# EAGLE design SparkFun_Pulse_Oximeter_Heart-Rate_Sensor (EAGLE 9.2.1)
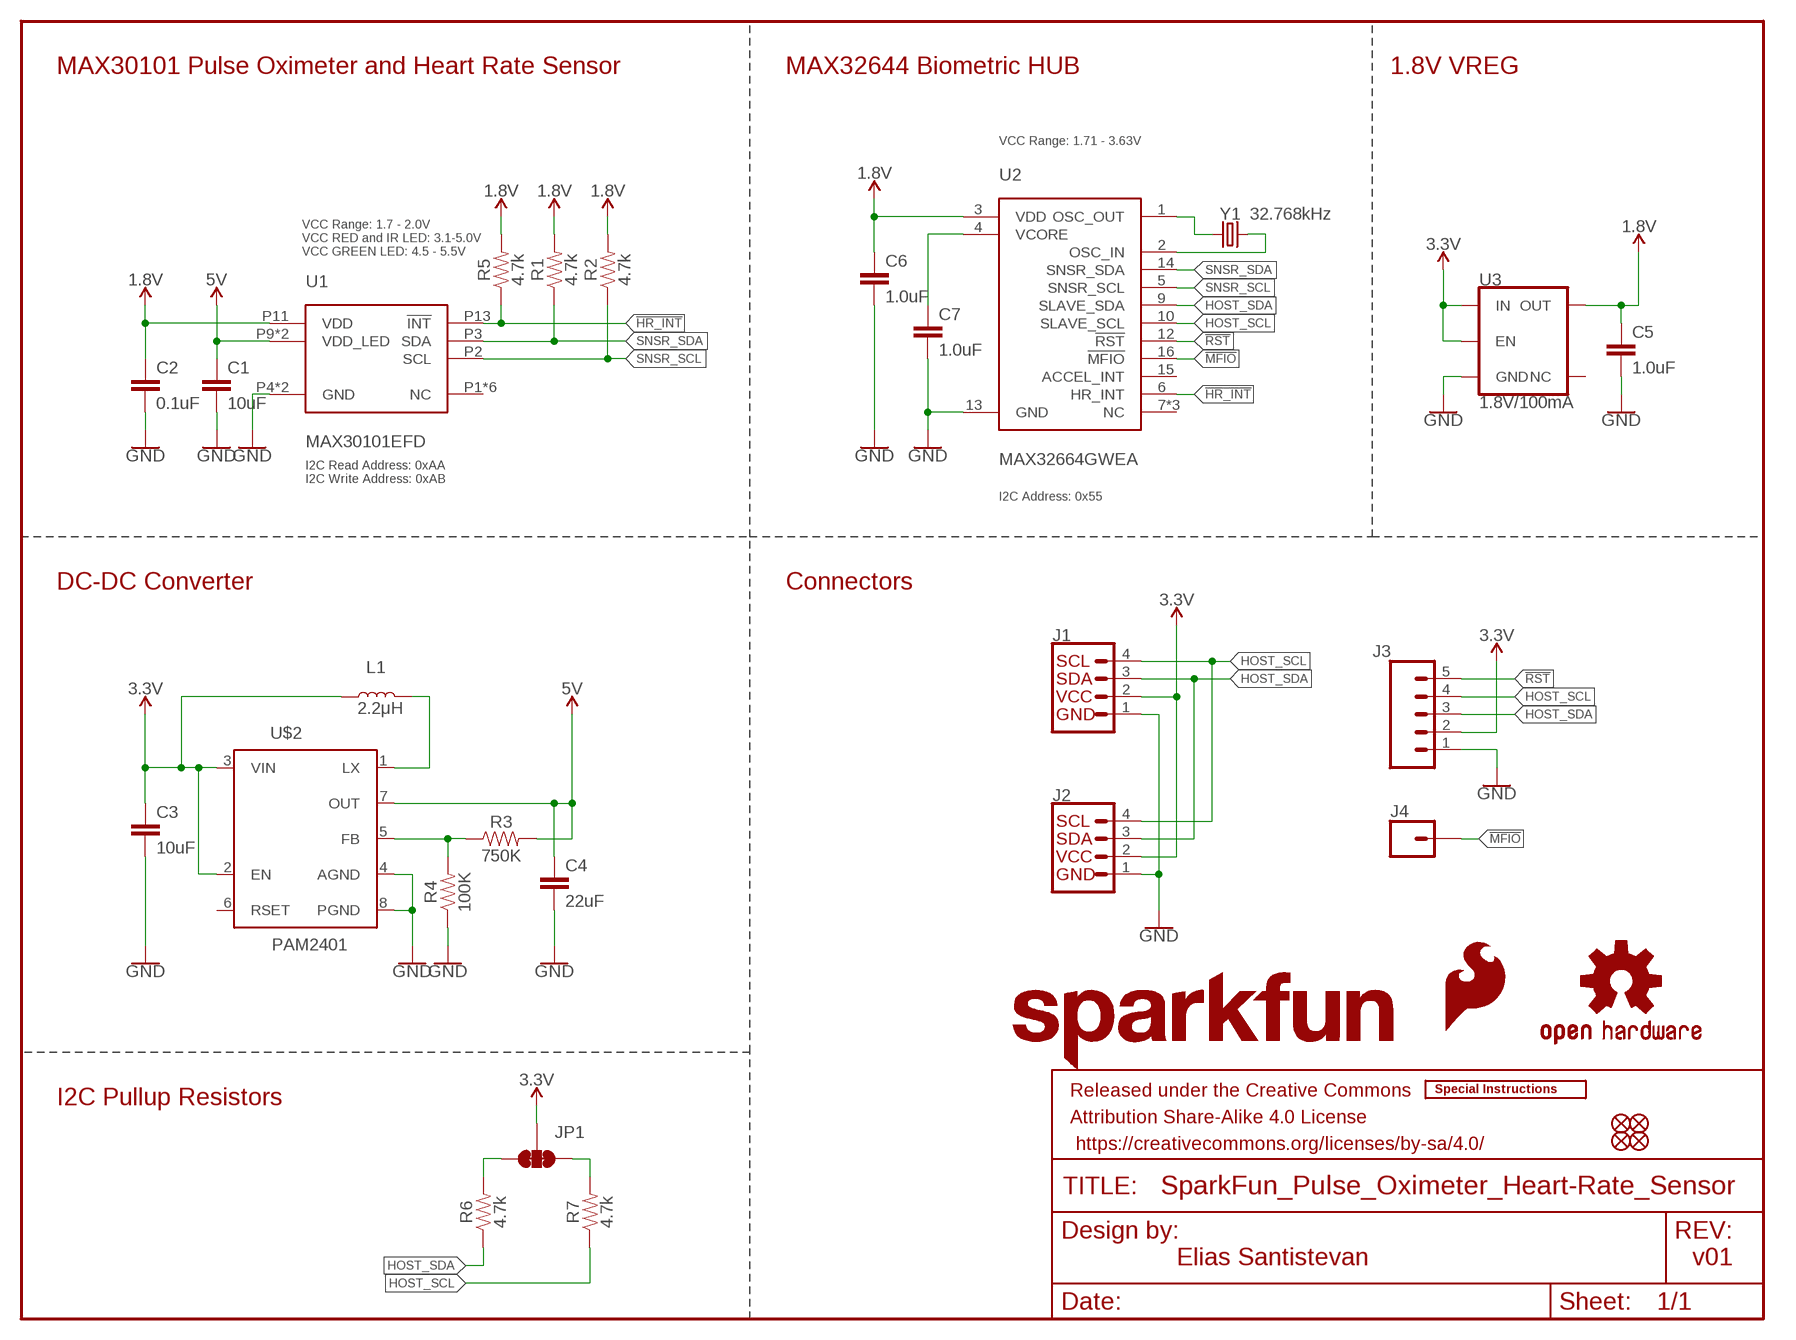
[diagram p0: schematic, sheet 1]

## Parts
C1  10uF  10UF-0603-6.3V-20%  [0603]
C2  0.1uF  0.1UF-0402-16V-10%  [0402]
C3  10uF  10UF-0603-6.3V-20%  [0603]
C4  22uF  22UF-0805-6.3V-20%  [0805]
C5  1.0uF  1.0UF-0603-16V-10%  [0603]
C6  1.0uF  1.0UF-0402-16V-10%  [0402]
C7  1.0uF  1.0UF-0402-16V-10%  [0402]
FD1  FIDUCIALUFIDUCIAL  [FIDUCIAL-MICRO]
FD2  FIDUCIALUFIDUCIAL  [FIDUCIAL-MICRO]
FD3  FIDUCIALUFIDUCIAL  [FIDUCIAL-MICRO]
FD4  FIDUCIALUFIDUCIAL  [FIDUCIAL-MICRO]
FRAME1  FRAME-LETTER  [CREATIVE_COMMONS]
J1  QWIIC_CONNECTORJS-1MM  [JST04_1MM_RA]
J2  QWIIC_CONNECTORJS-1MM  [JST04_1MM_RA]
J3  CONN_05NO_SILK  [1X05_NO_SILK]
J4  CONN_01PTH_NO_SILK_YES_STOP  [1X01_NO_SILK]
JP1  JUMPER-SMT_3_2-NC_TRACE_SILK  [SMT-JUMPER_3_2-NC_TRACE_SILK]
L1  2.2μH  2.2μH_SHIELDED_INDUCTOR  [0806]
LOGO1  SFE_LOGO_FLAME.1_INCH  [SFE_LOGO_FLAME_.1]
LOGO2  OSHW-LOGOMINI  [OSHW-LOGO-MINI]
LOGO3  SFE_LOGO_NAME.1_INCH  [SFE_LOGO_NAME_.1]
LOGO4  SPECIAL_INSTRUCTIONS-ORDERING  [ORDERING_INSTRUCTIONS]
R1  4.7k  4.7KOHM-0603-1/10W-1%  [0603]
R2  4.7k  4.7KOHM-0603-1/10W-1%  [0603]
R3  750K  750KOHM-0603-1/10W-1%  [0603]
R4  100K  100KOHM-0402-1/16W-1%  [0402]
R5  4.7k  4.7KOHM-0603-1/10W-1%  [0603]
R6  4.7k  4.7KOHM-0603-1/10W-1%  [0603]
R7  4.7k  4.7KOHM-0603-1/10W-1%  [0603]
U1  MAX30101EFD  [14_PIN_OESIP]
U2  MAX32664GWEA  [16_PIN_WLP]
U3  1.8V/100mA  V_REG_SP6214-1.8V  [SC70]
U$2  PAM2401  [MSOP8]
Y1  32.768kHz  CRYSTAL-32.768KHZSMD-3.2X1.5  [CRYSTAL-SMD-3.2X1.5MM]

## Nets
1.8V: C2.1 C5.1 C6.1 R1.2 R2.2 R5.2 U1.P11(VDD) U2.3(VDD) U3.5(OUT)
3.3V: C3.1 J1.2 J2.2 J3.2 JP1.2 L1.1 U3.1(IN) U3.3(EN) U$2.2(EN) U$2.3(VIN)
5V: C1.1 C4.1 R3.2 U1.P9(VDD_LED) U1.P10(VDD_LED) U$2.7(OUT)
!HR_INT: R5.1 U1.P13(!INT) U2.6(HR_INT)
!MFIO: J4.1 U2.16(!MFIO)
!RST: J3.5 U2.12(!RST)
GND: C1.2 C2.2 C3.2 C4.2 C5.2 C6.2 C7.2 J1.1 J2.1 J3.1 R4.1 U1.P4(GND) U1.P12(GND) U2.13(GND) U3.2(GND) U$2.4(AGND) U$2.8(PGND)
HOST_SCL: J1.4 J2.4 J3.4 R7.1 U2.10(SLAVE_SCL)
HOST_SDA: J1.3 J2.3 J3.3 R6.1 U2.9(SLAVE_SDA)
N$1: C7.1 U2.4(VCORE)
N$2: R3.1 R4.2 U$2.5(FB)
N$3: L1.2 U$2.1(LX)
N$4: JP1.3 R6.2
N$5: JP1.1 R7.2
N$6: U2.1(OSC_OUT) Y1.P$1
N$7: U2.2(OSC_IN) Y1.P$2
SNSR_SCL: R2.1 U1.P2(SCL) U2.5(SNSR_SCL)
SNSR_SDA: R1.1 U1.P3(SDA) U2.14(SNSR_SDA)
Unconnected: U1.P1(NC) U1.P5(NC) U1.P6(NC) U1.P7(NC) U1.P8(NC) U1.P14(NC) U2.7(NC) U2.8(NC) U2.11(NC) U2.15(ACCEL_INT) U3.4(NC) U$2.6(RSET)

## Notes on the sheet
- MAX30101 Pulse Oximeter and Heart Rate Sensor | MAX32644 Biometric HUB | 1.8V VREG
- VCC Range: 1.71 - 3.63V
- VCC Range: 1.7 - 2.0V
  VCC RED and IR LED: 3.1-5.0V
  VCC GREEN LED: 4.5 - 5.5V
- I2C Read Address: 0xAA
  I2C Write Address: 0xAB
- I2C Address: 0x55
- DC-DC Converter | Connectors
- I2C Pullup Resistors
- Elias Santistevan | v01

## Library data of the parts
C1 C3 = SparkFun-Capacitors:10UF: 10.0µF ceramic capacitors; PROD_ID: CAP-11015
C2 = SparkFun-Capacitors:0.1UF: 0.1µF ceramic capacitors; PROD_ID: CAP-12416
C4 = SparkFun-Capacitors:22UF: 22µF ceramic capacitors; PROD_ID: CAP-08402
C5 = SparkFun-Capacitors:1.0UF: 1µF ceramic capacitors; PROD_ID: CAP-00868
C6 C7 = SparkFun-Capacitors:1.0UF: 1µF ceramic capacitors; PROD_ID: CAP-12417
FD1-FD4 = SparkFun-Aesthetics:FIDUCIAL: Fiducial Alignment Points
FRAME1 = SparkFun-Aesthetics:FRAME-LETTER: Schematic Frame - Letter
J1 J2 = SparkFun-Connectors:QWIIC_CONNECTOR: SparkFun I2C Standard Qwiic Connector An SMD 1mm pitch JST connector makes it easy and quick (get it? Qwiic?) to connect I2C devices to each other. The Qwiic system enables fast and solderless connection between popular platforms and various sensors and actuators. We carry 200mm, 100mm, 50mm, and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; PROD_ID: CONN-13694
J3 = SparkFun-Connectors:CONN_05: Multi connection point. Often used as Generic Header-pin footprint for 0.1 inch spaced/style header connections On any of the 0.1 inch spaced packages, you can populate with these: Break Away Headers - Straight (PRT-00116) Break Away Male Headers - Right Angle (PRT-00553) Female Headers (PRT-00115)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
J4 = SparkFun-Connectors:CONN_01: Single connection point. Often used as Generic Header-pin footprint for 0.1 inch spaced/style header connections
JP1 = SparkFun-Jumpers:JUMPER-SMT_3_2-NC_TRACE: Normally closed trace jumper (2 of 2 connections) This jumper has a trace between all three pads so they are normally closed (NC). Use a razor knife to open the connection(s). For best results follow the IPC guidelines for cutting traces: Cutout at least 0.063 mm (0.005 in). Remove all loose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
L1 = SparkFun-Coils:2.2μH_SHIELDED_INDUCTOR: Murata 2.2uH Inductor; PROD_ID: NDUC-14257
LOGO1 = SparkFun-Aesthetics:SFE_LOGO_FLAME: SparkFun Flame Logo
LOGO2 = SparkFun-Aesthetics:OSHW-LOGO: Open-Source Hardware (OSHW) Logo
LOGO3 = SparkFun-Aesthetics:SFE_LOGO_NAME: SparkFun Font Logo
LOGO4 = SparkFun-Aesthetics:SPECIAL_INSTRUCTIONS: Special Ordering/Production Instructions Alert
R1 R2 R5-R7 = SparkFun-Resistors:4.7KOHM: 4.7kΩ resistor; PROD_ID: RES-07857
R3 = SparkFun-Resistors:750KOHM: 750Ω resistor; PROD_ID: RES-13768
R4 = SparkFun-Resistors:100KOHM: 100kΩ resistor; PROD_ID: RES-13495
U1 = SparkFun-IC-Special-Function:MAX30101EFD: MAX30101 High-Sensitivity Pulse Oximeter and Heart-Rate Sensor The MAX30101 is an integrated pulse oximetry and heart-rate monitor module. It includes internal LEDs, photodetectors, optical elements, and low-noise electronics with ambient light rejection. The MAX30101 provides a complete system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; PROD_ID: IC-14270
U2 = SparkFun-IC-Special-Function:MAX32664GWEA: Maxim MAX32664 Biometric Sensor Hub he MAX32664 is a sensor hub family with embedded firmware and algorithms for wearables. It seamlessly enables customer-desired sensor functionality, including communication with Maxim’s optical sensor solutions and delivering raw or calculated data to the outside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; PROD_ID: IC-14271
U3 = SparkFun-IC-Power:V_REG_SP6214: Voltage Regulator - SP6214 SP6214 Series SC-70-5 Micropower SC-70 100 mA CMOS LDO Regulator Datasheet SparkFun Products: MP3 Trigger SparkFun Particle Sensor Breakout; PROD_ID: VREG-08428
U$2 = SparkFun-IC-Power:PAM2401: PAM2401 - Boost PMIC Specifications: Up to 1A output current 0.9V to 4.75V Input Range 2.5V to 5.0V Adjustable Output Voltage Datasheet (Diodes inc.); PROD_ID: IC-13769
Y1 = SparkFun-Clocks:CRYSTAL-32.768KHZ: 32.768kHz Crystal; PROD_ID: XTAL-13062

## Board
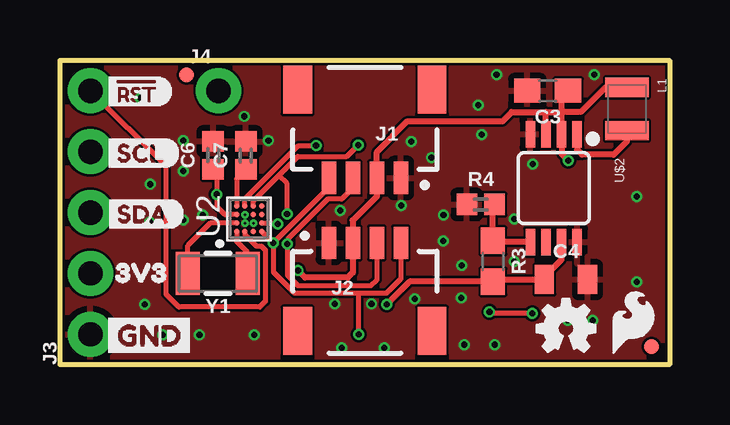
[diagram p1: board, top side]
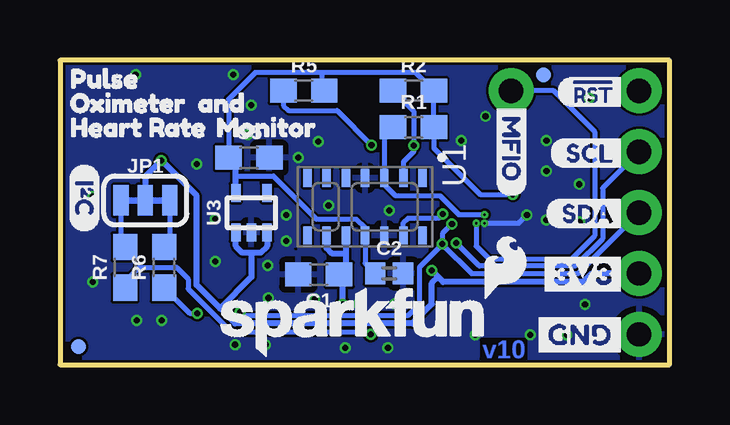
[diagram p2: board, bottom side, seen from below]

Size 25.4 x 12.7 mm. Coordinates in mm from the lower left corner, seen from the top.
Outline: 0,0 0,12.7 25.4,12.7 25.4,0 0,0
Copper layers (1*16): Top 0.035mm / dielectric 1.5mm / Bottom 0.035mm
Design rules "SparkFun-2-layer-FAB-LIMIT *": minimum track width 4mil, minimum drill 4mil, track to track 4mil, track to pad 4mil, pad to pad 4mil, via to via 4mil, smd to smd 4mil, copper to edge 4mil, drill to drill 4mil, minimum pad ring 5mil, minimum via ring 4mil, stop-mask expansion 4mil, vias tented up to drill 25mil, thermal gap 10mil

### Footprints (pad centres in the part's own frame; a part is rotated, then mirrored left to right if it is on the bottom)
0603 = smd 1.1 x 1: 1 -0.85,0; 2 0.85,0
0402 = smd 0.85 x 0.9: 1 -0.58,0; 2 0.58,0
0805 = smd 0.8 x 1.2: 1 -0.9,0; 2 0.9,0
FIDUCIAL-MICRO = smd 0.635 x 0.635: 1 0,0
JST04_1MM_RA = smd 0.6 x 1.35: 1 -1.5,0; 2 -0.5,0; 3 0.5,0; 4 1.5,0 | smd 1.2 x 2: NC1 2.8,-3.675; NC2 -2.8,-3.675
1X05_NO_SILK = drill 1.016 pad 1.88: 1 0,0; 2 2.54,0; 3 5.08,0; 4 7.62,0; 5 10.16,0
1X01_NO_SILK = drill 1.016 pad 1.88: 1 0,0
SMT-JUMPER_3_2-NC_TRACE_SILK = smd 0.635 x 1.27: 1 -1.016,0; 2 0,0; 3 1.016,0
0806 = smd 0.8 x 1.8: 1 -0.9,0; 2 0.9,0
14_PIN_OESIP = smd 0.75 x 0.35: P1 -1.193,2.409; P2 -1.193,1.609; P3 -1.193,0.809; P4 -1.193,0.009; P5 -1.193,-0.791; P6 -1.193,-1.591; P7 -1.193,-2.391; P8 1.207,-2.391; P9 1.207,-1.591; P10 1.207,-0.791; P11 1.207,0.009; P12 1.207,0.809; P13 1.207,1.609; P14 1.207,2.409
16_PIN_WLP = smd 0.22 x 0.22: 1 -0.532,0.518; 2 -0.182,0.518; 3 0.168,0.518; 4 0.518,0.518; 5 0.518,0.168; 6 0.518,-0.182; 7 0.518,-0.532; 8 0.168,-0.532; 9 -0.182,-0.532; 10 -0.532,-0.532; 11 -0.532,-0.182; 12 -0.532,0.168; 13 -0.182,0.168; 14 0.168,0.168; 15 0.168,-0.182; 16 -0.182,-0.182
SC70 = smd 0.4 x 0.75: 1 -0.65,-0.825; 2 0,-0.825; 3 0.65,-0.825; 4 0.65,0.825; 5 -0.65,0.825
MSOP8 = smd 0.4 x 1.1: 1 -0.975,-2.25; 2 -0.325,-2.25; 3 0.325,-2.25; 4 0.975,-2.25; 5 0.975,2.25; 6 0.325,2.25; 7 -0.325,2.25; 8 -0.975,2.25
CRYSTAL-SMD-3.2X1.5MM = smd 1 x 1.8: P$1 -1.25,0; P$2 1.25,0

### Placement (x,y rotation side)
C1  14.62,3.76 180 bottom
C2  11.68,3.81 0 bottom
C3  20.32,11.43 180 top
C4  21.08,3.56 0 top
C5  17.53,8.64 0 bottom
C6  6.38,8.74 90 top
C7  7.75,8.74 90 top
FD1  5.26,12.08 0 bottom
FD2  5.27,12.08 0 top
FD3  24.64,0.76 0 bottom
FD4  24.64,0.76 0 top
FRAME1  not placed on the board
J1  12.7,7.8 180 top
J2  12.7,5.08 0 top
J3  1.27,1.27 90 top
J4  6.6,11.43 0 top
JP1  21.84,6.86 0 bottom
L1  23.62,10.67 270 top
LOGO1  23.88,1.78 0 top
LOGO2  21.08,1.52 0 top
LOGO3  13.21,1.78 0 bottom
LOGO4  not placed on the board
R1  10.67,9.91 0 bottom
R2  10.67,11.43 0 bottom
R3  18.03,4.32 270 top
R4  17.53,6.69 0 top
R5  15.24,11.43 0 bottom
R6  21.06,4.06 90 bottom
R7  22.68,4.06 90 bottom
U1  12.7,6.6 270 bottom
U2  7.87,6.1 90 top
U3  17.42,6.35 0 bottom
U$1  [I_SUPER2_C-()-03]  24.38,8.38 270 bottom
U$2  20.57,7.37 180 top
U$3  [GND-03]  5.88,1.25 0 bottom
U$4  [SCL0]  1.68,8.83 0 top
U$5  [GND-03]  1.6,1.23 0 top
U$6  [#RST0]  1.56,11.41 0 top
U$7  [MFIO0]  6.59,11.08 270 bottom
U$8  [#RST0]  4.82,11.38 0 bottom
U$9  [SCL0]  5,8.83 0 bottom
U$10  [SDA0]  5.18,6.31 0 bottom
U$11  [GND-03]  1.63,1.25 180 bottom
U$12  [3V3-03]  5.67,3.78 0 bottom
U$13  [3V3-TEXT]  1.61,3.84 0 top
U$14  [OXIMETER0]  25.65,10.92 0 bottom
U$15  [HEART_RATE0]  25.65,9.91 0 bottom
U$16  [MONITOR0]  19.56,9.91 0 bottom
U$17  [PULSE0]  25.65,11.94 0 bottom
U$18  [AND0]  20.32,10.92 0 bottom
U$19  [SFE_LOGO_FLAME_.1]  6.86,4.06 0 bottom
U$20  [SDA0]  1.68,6.29 0 top
Y1  6.58,3.81 180 top

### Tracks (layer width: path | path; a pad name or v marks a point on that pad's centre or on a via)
1.8V  (via drill 0.25)
  Top 0.203: C6.1 6.53,8.02 v6.53,7.11 6.53,6.6 6.87,6.26 U2.3
  Bottom 0.203: C2.1 12.69,4.24 U1.P11 12.69,5.71 13.05,6.07 14.7,6.07 16.51,7.87 18.07,7.87 | 14.48,12.19 10.58,12.19 R2.2 R1.2 9.82,9.04 7.89,7.11 v6.53,7.11 | 14.48,12.19 17.27,12.19 18.38,11.09 C5.1 | R5.2 14.48,11.52 14.48,12.19
  Bottom 0.254: U3.5 18.07,7.87 18.07,8.33 C5.1
3.3V  (via drill 0.25)
  Top 0.254: 20.9,10.54 U$2.2 20.9,8.8 v21.18,8.52 | 20.9,10.54 20.9,11.16 C3.1 | L1.1 22.72,11.57 21.7,10.54 20.9,10.54 | 20.24,10.54 18.82,10.54 18.44,10.16 14.48,10.16 13.2,8.88 J1.2 13.2,7.03 12.19,6.02 J2.2 12.2,3.84 11.99,3.64 10.22,3.64 v9.92,3.94 | 20.24,10.54 20.9,10.54 | U$2.3 20.25,10.54 20.24,10.54
  Bottom 0.254: J3.2 3.24,3.81 3.59,3.46 9.43,3.46 9.65,3.67 | 9.65,3.67 v9.92,3.94 | JP1.2 21.84,7.85 v21.18,8.52 21.17,8.52 19.71,7.06 19.71,3.33 18.73,2.35 | 18.73,2.35 18.11,1.73 10.72,1.73 9.91,2.54 9.91,3.41 9.65,3.67 | U3.3 16.77,4.94 17.05,4.67 17.42,4.67 | 17.42,4.67 17.8,4.67 18.07,4.94 U3.1 | 17.42,4.67 17.42,3.66 18.73,2.35
5V  (via drill 0.25)
  Top 0.254: 20.07,3.56 18.12,3.56 R3.2 14.57,3.47 v13.61,2.52 | 20.07,3.56 C4.1 | 20.07,3.56 20.9,4.39 U$2.7
  Bottom 0.254: v13.61,2.52 13.61,3.6 | 13.61,3.6 13.61,3.8 13.49,3.92 13.49,4.65 | 13.61,3.6 C1.1 | U1.P10 13.49,4.65 | U1.P9 14.29,4.87 14.07,4.65 13.49,4.65
!HR_INT  (via drill 0.25)
  Top 0.203: v12.42,9.17 11.94,8.69 9.91,8.69 9.12,7.9 | 9.12,7.9 8.06,6.84 U2.6 | v9.46,6.29 9.46,7.56 9.12,7.9
  Bottom 0.203: U1.P13 11.09,5.93 10.9,6.12 9.63,6.12 v9.46,6.29 | R5.1 16.09,10.82 15.88,10.6 13.86,10.6 v12.42,9.17
!MFIO  (via drill 0.1)
  Top 0.203: U2.16
  Bottom 0.203: U2.16 8.06,4.96 7.52,4.42 4.07,4.42 3.1,5.39 3.1,9.7 4.83,11.43 J4.1
  other vias: 8.06,5.91
!RST
  Top 0.203: J3.5 4.42,8.28 4.42,2.95 4.95,2.41 8.33,2.41 8.56,2.64 8.56,4.78 8.39,4.95 8.18,4.95 7.71,5.43 U2.12
GND  (via drill 0.1, 0.25)
  Top 0.203: U2.13 | U2.13
  Bottom 0.203: U2.13 6.28,5.91 v5.94,6.25
  other vias: 8.69,9.35 7.67,10.36 5.13,9.35 7.71,5.91 11.67,6.43 15.98,6.26 15.97,5.16 19.7,8.37 22.2,1.86 21.16,1.86 3.75,5.95 3.77,7.53 5.81,1.25 8.1,1.25 5.13,8.08 5.13,6.05 14.78,2.74 16.71,2.79 13.51,0.71 11.73,0.71 16.74,4.14 14.63,9.3 15.48,8.64 17.43,10.83 18.19,12.1 24.03,7.02 24.03,3.46 4.29,1.25 3.53,2.52 17.58,9.6 16.84,0.84 18.11,0.84 3.35,11.13 14.21,6.64 11.46,2.54 12.98,2.54 18.93,6.09 18.93,4.31 22.25,12.1
  pour Top: 0,12.7 0,0 25.4,0 25.4,12.7
  pour Bottom: 0,12.7 0,0 25.4,0 25.4,12.7
HOST_SCL  (via drill 0.25)
  Top 0.203: J2.4 14.2,3.58 13.61,3 12.45,3 | J1.4 11.2,7.39 v8.89,5.08 | 12.45,3 9.76,3 8.89,3.87 v8.89,5.08 | v12.45,1.27 12.45,3 | U2.10 v8.89,5.08
  Bottom 0.203: J3.4 2.79,7.37 2.79,5.26 3.94,4.12 7.92,4.12 v8.89,5.08 | R7.1 22.68,3.48 22.1,4.06 20.54,4.06 20.07,3.59 20.07,3.17 18.26,1.37 12.55,1.37 v12.45,1.27
HOST_SDA  (via drill 0.25)
  Top 0.203: J2.3 13.2,3.55 12.95,3.3 9.91,3.3 9.47,3.74 v9.47,5.03 9.47,5.23 11.15,6.91 11.73,6.91 12.2,7.37 J1.3 | v19.68,2.15 17.95,2.15 v17.89,2.21 | v9.07,5.87 9.03,5.91 U2.9
  Bottom 0.203: v9.07,5.87 9.47,5.47 v9.47,5.03 | v9.47,5.03 8.25,3.81 3.81,3.81 J3.3 | R6.1 19.99,2.15 v19.68,2.15 | v17.89,2.21 17.75,2.07 10.89,2.07 10.41,2.54 10.41,4.08 v9.47,5.03
N$1
  Top 0.203: C7.1 7.36,7.77 U2.4
N$2
  Top 0.254: U$2.5 18.09,5.12 R3.1 18.03,6.61 R4.2
N$3
  Top 0.254: U$2.1 21.55,8.97 21.76,8.77 23.07,8.77 23.62,9.32 L1.2
N$4
  Bottom 0.203: JP1.3 20.83,5.14 R6.2
N$5
  Bottom 0.203: JP1.1 22.86,5.09 R7.2
N$6
  Top 0.203: Y1.P$1 7.83,3.91 7.8,3.94 7.8,4.7 7.36,5.14 U2.1 | U2.1
N$7
  Top 0.203: Y1.P$2 5.33,4.97 6.27,5.91 U2.2
SNSR_SCL  (via drill 0.25)
  Top 0.203: v10.67,9.14 9.93,9.14 7.71,6.92 U2.5
  Bottom 0.203: R2.1 10.67,10.58 v10.67,9.14 10.67,8.89 11.09,8.47 U1.P2
SNSR_SDA  (via drill 0.1)
  Top 0.203: U2.14
  Bottom 0.203: R1.1 11.89,9.53 U1.P3 11.89,7.51 11.43,7.05 9.58,7.05 8.79,6.26 U2.14
  other vias: 7.71,6.26

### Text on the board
Bottom: v10
Measures: Measurments in Inches
tDocu: Elias Santistevan | Via on Pad for small BGA

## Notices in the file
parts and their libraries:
SparkFun-Aesthetics: Licensing: Creative Commons ShareAlike 4.0 International - https://creativecommons.org/licenses/by-sa/4.0
SparkFun-Aesthetics: Released under the Creative Commons Attribution Share-Alike 4.0 License
SparkFun-Aesthetics: https://creativecommons.org/licenses/by-sa/4.0
